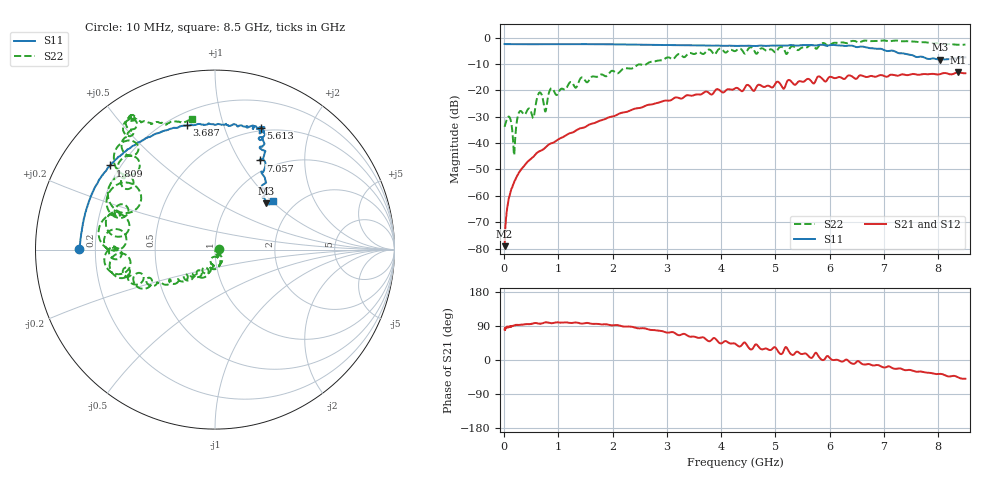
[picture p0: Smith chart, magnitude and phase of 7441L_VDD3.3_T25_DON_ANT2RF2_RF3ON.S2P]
!Agilent Technologies,E5071C,MY46417908,A.11.23
!Date: Mon May 03 19:54:22 2021
!Data & Calibration Information:
!Freq	S11:SOLT2(ON)	S21:SOLT2(ON)	S12:SOLT2(ON)	S22:SOLT2(ON)
!PortZ  Port1:50+j0  Port2:50+j0
!Above PortZ is port z conversion or system Z0 setting when saving the data.
!When reading, reference impedance value at option line is always used.
# Hz S dB R 50
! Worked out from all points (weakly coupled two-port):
!   1601 points, 10 MHz to 8.5 GHz, reference 50 ohm
!   highest |S21| = -13.21 dB at 8.367 GHz (marker M1); lowest = -79.1 dB at 10 MHz (marker M2)
!   lowest |S11| = -8.3 dB at 8.028 GHz (marker M3), VSWR 2.25, Z = 73.7 + j44.7 ohm
!   |S11| at or under -10 dB: nowhere
!   |S22| runs from -44.6 to -1.1 dB; largest |S21 - S12| = 0.0035
!   S11 on the Smith chart (normalised r, x): 10 MHz: 0.14, +0.00; 1.809 GHz: 0.16, +0.34; 3.687 GHz: 0.27, +0.76; 5.613 GHz: 0.47, +1.33; 7.057 GHz: 0.86, +1.23; 8.5 GHz: 1.55, +1.02
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1e7  -2.42 179.7  -79.11 80.5  -79.10 77.0  -33.81 2.9
9.49e7  -2.47 177.5  -60.50 86.8  -60.52 88.5  -30.02 -42.3
1.851062e8  -2.49 175.2  -54.88 90.8  -54.87 91.4  -44.58 -37.2
2.593938e8  -2.49 173.3  -51.85 92.4  -51.75 93.0  -29.31 -20.3
3.0715e8  -2.51 172.2  -50.26 93.2  -50.24 92.5  -27.83 -51.0
5.300125e8  -2.49 166.7  -45.36 96.0  -45.34 95.7  -30.44 -75.2
6.520562e8  -2.49 164.0  -43.08 96.0  -43.12 95.7  -20.82 -80.4
7.634875e8  -2.49 161.3  -41.66 99.5  -41.64 99.3  -28.02 -87.3
8.643062e8  -2.48 159.1  -40.11 97.2  -40.13 96.9  -19.27 -89.1
9.757375e8  -2.47 156.9  -38.92 99.3  -38.90 99.4  -21.71 -100.9
1.426769e9  -2.46 148.4  -34.32 96.1  -34.29 96.2  -15.12 -117.7
1.808819e9  -2.51 141.2  -31.27 93.9  -31.24 94.0  -13.99 -133.4
2.843538e9  -2.75 121.0  -24.66 77.5  -24.68 77.5  -8.68 -149.9
3.687231e9  -2.97 102.7  -20.69 58.7  -20.71 58.7  -6.07 -164.0
4.255e9  -3.14 90.5  -19.24 43.2  -19.26 43.0  -5.12 179.7
5.6134e9  -2.81 69.5  -15.68 9.6  -15.67 10.0  -3.22 141.5
5.671769e9  -2.88 70.1  -16.85 5.9  -16.84 5.9  -2.81 135.2
7.0567e9  -5.08 63.0  -14.84 -17.8  -14.80 -17.6  -1.23 121.3
7.088538e9  -5.04 63.6  -14.45 -16.6  -14.43 -16.3  -1.38 121.9
8.027744e9  -8.30 42.2  -13.90 -36.6  -13.84 -37.0  -2.21 113.9
8.367344e9  -7.87 40.1  -13.21 -46.0  -13.10 -45.7  -2.72 104.2
8.5e9  -7.47 39.8  -13.50 -49.5  -13.39 -49.1  -2.64 100.0
